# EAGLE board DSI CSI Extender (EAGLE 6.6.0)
REV: A
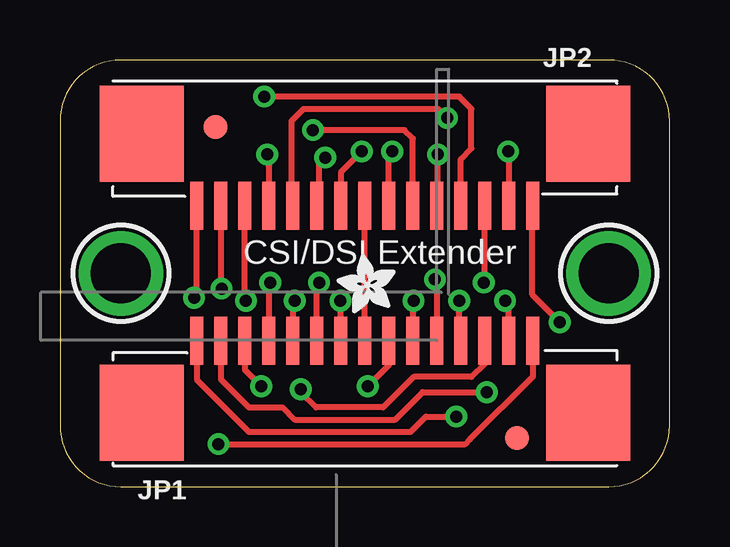
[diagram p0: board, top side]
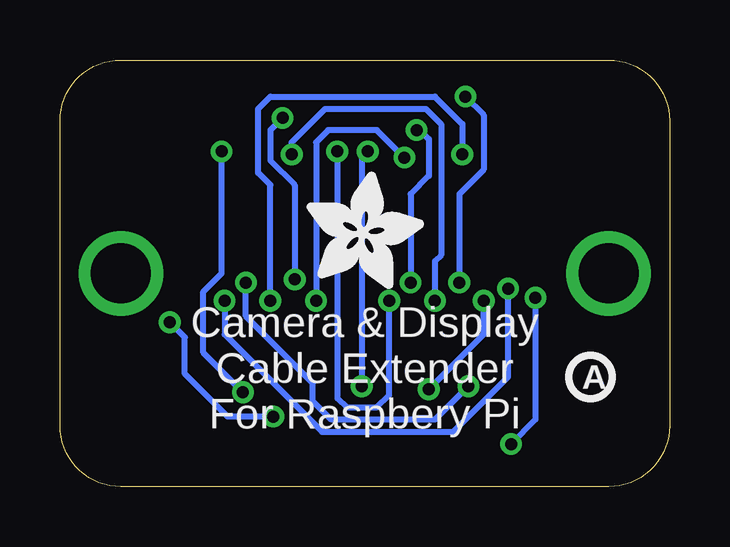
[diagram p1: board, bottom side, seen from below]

Size 25.4 x 17.78 mm. Coordinates in mm from the lower left corner, seen from the top.
Outline: 0,15.24 0,2.54 arc90 2.54,0 22.86,0 arc90 25.4,2.54 25.4,15.24 arc90 22.86,17.78 2.54,17.78 arc90 0,15.24
Copper layers (1*16): Top 0.035mm / dielectric 1.5mm / Bottom 0.035mm
Design rules "adafruit *": minimum track width 8mil, minimum drill 16mil, track to track 8mil, track to pad 8mil, pad to pad 8mil, via to via 8mil, smd to smd 8mil, copper to edge 10mil, drill to drill 8mil, minimum pad ring 10mil, minimum via ring 8mil, stop-mask expansion 4mil, vias tented up to drill 20mil, thermal gap 10mil

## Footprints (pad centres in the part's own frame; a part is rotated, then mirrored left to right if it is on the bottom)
FIDUCIAL_1MM = smd 1 x 1: 1 0,0
FPC_15PIN_1.0MM = smd 0.55 x 2: 1 -7,1; 2 -6,1; 3 -5,1; 4 -4,1; 5 -3,1; 6 -2,1; 7 -1,1; 8 0,1; 9 1,1; 10 2,1; 11 3,1; 12 4,1; 13 5,1; 14 6,1; 15 7,1 | smd 3.5 x 4: M1 -9.3,-2; M2 9.3,-2
MOUNTINGHOLE_2.5_PLATED = drill 2.5 pad 3.2: P$1 0,0

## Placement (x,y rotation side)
FID1  FIDUCIAL_1MM  [FIDUCIAL_1MM]  19.05,2.03 0 top
FID2  FIDUCIAL_1MM  [FIDUCIAL_1MM]  6.48,14.99 0 top
JP1  [FPC_15PIN_1.0MM]  12.7,5.08 0 top
JP2  [FPC_15PIN_1.0MM]  12.7,12.7 180 top
U$2  MOUNTINGHOLE2.5  [MOUNTINGHOLE_2.5_PLATED]  2.54,8.89 0 top
U$3  MOUNTINGHOLE2.5  [MOUNTINGHOLE_2.5_PLATED]  22.86,8.89 0 top
U$4  [ADAFRUIT_2.5MM]  13.97,7.24 90 top
U$5  [ADAFRUIT_5MM]  15.11,8.26 0 bottom
U$6  [PCBFEAT-REV-040]  3.3,4.57 0 bottom

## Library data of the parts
FID1 FID2 U$2 U$3 = microbuilder; BOM: EXCLUDE
JP1 JP2 U$4-U$6 = microbuilder

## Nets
N$1: JP1.1 JP2.1
N$2: JP1.2 JP2.2
N$3: JP1.3 JP2.3
N$4: JP1.4 JP2.4
N$5: JP1.5 JP2.5
N$6: JP1.6 JP2.6
N$7: JP1.7 JP2.7
N$8: JP1.8 JP2.8
N$9: JP1.9 JP2.9
N$10: JP1.10 JP2.10
N$11: JP1.11 JP2.11
N$12: JP1.12 JP2.12
N$13: JP1.13 JP2.13
N$14: JP1.14 JP2.14
N$15: JP1.15 JP2.15

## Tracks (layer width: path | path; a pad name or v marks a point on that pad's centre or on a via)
N$1  (via drill 0.5)
  Top 0.254: JP1.1 5.7,4.46 7.87,2.29 14.61,2.29 15.24,2.92 v16.51,2.92 | v20.83,6.86 19.68,8 19.68,11.69 JP2.1
  Bottom 0.254: v16.51,2.92 18.41,2.92 20.19,4.7 20.19,6.22 v20.83,6.86
N$2  (via drill 0.5)
  Top 0.254: JP1.2 6.7,4.48 7.87,3.3 9.27,3.3 9.78,2.79 13.97,2.79 15.11,3.94 v17.78,3.94 | v18.67,13.97 18.7,13.94 JP2.2
  Bottom 0.254: v17.78,3.94 19.43,5.59 19.43,8.13 18.67,8.89 v18.67,13.97
N$3  (via drill 0.5)
  Top 0.254: JP1.3 7.7,4.87 v8.38,4.19 | JP2.3 17.7,8.56 v17.65,8.51
  Bottom 0.254: v8.38,4.19 9.78,2.79 14.1,2.79 14.86,3.56 14.86,4.32 17.65,7.11 v17.65,8.51
N$4  (via drill 0.5)
  Top 0.254: JP2.4 16.7,13.65 17.14,14.1 17.14,15.75 16.64,16.26 v8.51,16.26 | v8.76,8.51 8.7,8.45 JP1.4
  Bottom 0.254: v8.51,16.26 7.75,15.49 7.75,13.21 8.76,12.19 v8.76,8.51
N$5  (via drill 0.5)
  Top 0.254: JP2.5 15.75,11.75 v15.75,13.84 | v9.78,7.75 9.7,7.67 JP1.5
  Bottom 0.254: v15.75,13.84 15.75,14.35 14.35,15.75 10.16,15.75 9.53,15.11 9.53,9.65 9.78,9.4 v9.78,7.75
N$6  (via drill 0.5)
  Top 0.254: JP2.6 14.7,14.51 14.35,14.86 v10.54,14.86 | JP1.6 10.7,8.41 v10.79,8.51
  Bottom 0.254: v10.54,14.86 10.54,14.99 10.03,14.48 10.03,12.95 10.79,12.19 v10.79,8.51
N$7  (via drill 0.5)
  Top 0.254: JP2.7 13.7,13.83 v13.84,13.97 | JP1.7 11.7,7.73 v11.68,7.75
  Bottom 0.254: v13.84,13.97 13.84,3.68 13.46,3.3 12.19,3.3 11.68,3.81 v11.68,7.75
N$8
  Top 0.254: JP1.8 JP2.8
N$9  (via drill 0.5)
  Top 0.254: JP1.9 13.7,5.06 v12.83,4.19 | v12.57,13.97 11.7,13.1 JP2.9
  Bottom 0.254: v12.57,13.97 12.83,13.72 v12.83,4.19
N$10  (via drill 0.5)
  Top 0.254: JP2.10 10.79,11.79 10.79,13.46 v11.05,13.72 | v14.73,7.75 14.7,7.71 JP1.10
  Bottom 0.254: v11.05,13.72 12.19,14.86 14.22,14.86 14.73,14.35 v14.73,7.75
N$11  (via drill 0.5)
  Top 0.254: JP2.11 9.65,11.75 9.65,15.24 10.16,15.75 15.75,15.75 v16.13,15.37 | v15.62,8.64 15.7,8.56 JP1.11
  Bottom 0.254: v16.13,15.37 16.64,14.86 16.64,13.59 15.62,12.57 v15.62,8.64
N$12  (via drill 0.5)
  Top 0.254: JP1.12 16.64,6.14 v16.64,7.75 | v8.64,13.84 8.7,13.78 JP2.12
  Bottom 0.254: v16.64,7.75 16.64,12.57 17.14,13.08 17.14,15.75 16.64,16.26 9.78,16.26 8.64,15.11 v8.64,13.84
N$13  (via drill 0.5)
  Top 0.254: JP1.13 17.7,5.13 17.14,4.57 14.73,4.57 13.46,3.3 10.67,3.3 10.03,3.94 v10.03,4.06 | v7.75,7.75 7.7,7.79 JP2.13
  Bottom 0.254: v10.03,4.06 7.75,6.35 v7.75,7.75
N$14  (via drill 0.5)
  Top 0.254: JP1.14 18.7,7.59 v18.54,7.75 | JP2.14 6.7,8.29 v6.73,8.26
  Bottom 0.254: v18.54,7.75 18.54,6.35 14.48,2.29 9.02,2.29 6.73,4.57 v6.73,8.26
N$15  (via drill 0.5)
  Top 0.254: JP1.15 19.7,4.59 17.08,1.97 16.89,1.78 v6.6,1.78 | JP2.15 5.7,7.99 v5.59,7.87
  Bottom 0.254: v5.59,7.87 5.59,2.79 v6.6,1.78

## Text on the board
tPlace: CSI/DSI Extender
bPlace: Camera & Display / Cable Extender / For Raspbery Pi

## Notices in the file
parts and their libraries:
microbuilder: This work is placed in the public domain, and may be freely used for commercial and non-commercial work with the following conditions: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
